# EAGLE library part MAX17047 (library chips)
1-Cell Fuel Gauge with ModelGauge m3
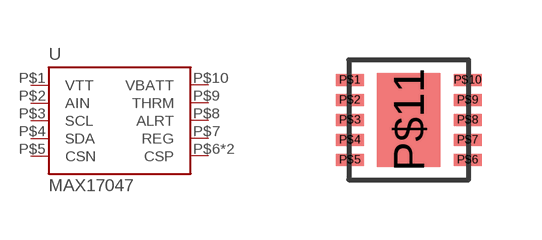
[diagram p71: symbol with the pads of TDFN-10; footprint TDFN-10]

Designator prefix U

## MAX17047 (MOUSER: 700-MAX17047G+)  [TDFN-10]
P$1  VTT
P$2  AIN
P$3  SCL
P$4  SDA
P$5  CSN
P$6  CSP
P$7  REG
P$8  ALRT
P$9  THRM
P$10  VBATT
P$11  CSP

## Footprint TDFN-10 (pad centres in mm)
smd 0.7 x 0.3: P$1 -1.475,1; P$2 -1.475,0.5; P$3 -1.475,0; P$4 -1.475,-0.5; P$5 -1.475,-1; P$6 1.475,-1; P$7 1.475,-0.5; P$8 1.475,0; P$9 1.475,0.5; P$10 1.475,1
smd 1.58 x 2.35: P$11 0,0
